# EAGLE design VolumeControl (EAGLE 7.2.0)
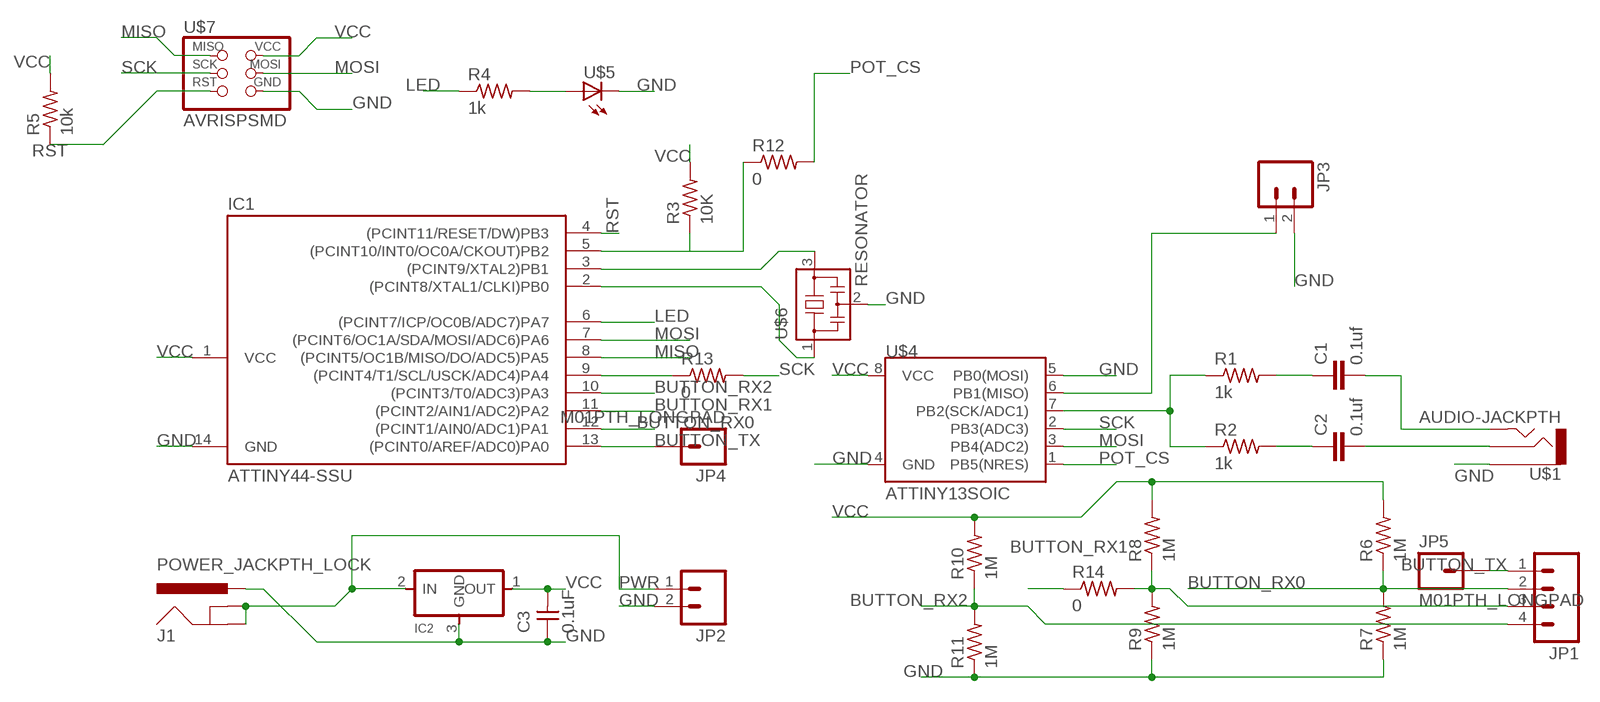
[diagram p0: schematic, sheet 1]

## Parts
C1  0.1uf  CAP1206  [1206]
C2  0.1uf  CAP1206  [1206]
C3  0.1uF  UNPOLARIZED_CAPACITOR1206  [1206]
IC1  ATTINY44-SSU  [SOIC14]
IC2  REGULATORSOT23  [SOT23]
J1  POWER_JACKPTH_LOCK  [POWER_JACK_PTH_LOCK]
JP1  M04SMD  [1X04-SMD]
JP2  M02LOCK_LONGPADS  [1X02_LOCK_LONGPADS]
JP3  M02LOCK_LONGPADS  [1X02_LOCK_LONGPADS]
JP4  M01PTH_LONGPAD  [1X01_LONGPAD]
JP5  M01PTH_LONGPAD  [1X01_LONGPAD]
R1  1k  RESISTOR1206  [1206]
R2  1k  RESISTOR1206  [1206]
R3  10K  RESISTOR1206  [1206]
R4  1k  RESISTOR1206  [1206]
R5  10k  RESISTOR1206  [1206]
R6  1M  RESISTOR1206  [1206]
R7  1M  RESISTOR1206  [1206]
R8  1M  RESISTOR1206  [1206]
R9  1M  RESISTOR1206  [1206]
R10  1M  RESISTOR1206  [1206]
R11  1M  RESISTOR1206  [1206]
R12  0  RESISTOR1206  [1206]
R13  0  RESISTOR1206  [1206]
R14  0  RESISTOR1206  [1206]
U$1  AUDIO-JACKPTH  [AUDIO-JACK]
U$4  ATTINY13SOIC  [SO08]
U$5  LED1206  [1206]
U$6  RESONATOR  [EFOBM]
U$7  AVRISPSMD  [2X03SMD]

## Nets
BUTTON_RX0: IC1.12((PCINT1/AIN0/ADC1)PA1) JP1.2 R6.1 R7.2
BUTTON_RX1: IC1.11((PCINT2/AIN1/ADC2)PA2) JP1.3 R8.1 R9.2 R14.1 R14.2
BUTTON_RX2: IC1.10((PCINT3/T0/ADC3)PA3) JP1.4 R10.1 R11.2
BUTTON_TX: IC1.13((PCINT0/AREF/ADC0)PA0) JP1.1 JP4.1 JP5.1
GND: C3.1 IC1.14(GND) IC2.3(GND) J1.PWR JP2.2 JP3.2 R7.1 R9.1 R11.1 U$1.1 U$4.4(GND) U$4.5(PB0(MOSI)) U$5.2(C) U$6.2 U$7.6(GND)
LED: IC1.6((PCINT7/ICP/OC0B/ADC7)PA7) R4.1
MISO: IC1.8((PCINT5/OC1B/MISO/DO/ADC5)PA5) U$7.1(MISO)
MOSI: IC1.7((PCINT6/OC1A/SDA/MOSI/ADC6)PA6) U$4.3(PB4(ADC2)) U$7.4(MOSI)
N$8: C2.2 U$1.2
N$9: C1.2 U$1.5
N$10: C1.1 R1.2
N$11: C2.1 R2.2
N$12: R1.1 R2.1 U$4.7(PB2(SCK/ADC1))
N$13: JP3.1 U$4.6(PB1(MISO))
N$14: R4.2 U$5.1(A)
N$15: IC1.3((PCINT9/XTAL2)PB1) U$6.3
N$16: IC1.2((PCINT8/XTAL1/CLKI)PB0) U$6.1
POT_CS: IC1.5((PCINT10/INT0/OC0A/CKOUT)PB2) R3.1 R12.1 R12.2 U$4.1(PB5(NRES))
PWR: IC2.2(IN) J1.GND J1.GNDBREAK JP2.1
RST: IC1.4((PCINT11/RESET/DW)PB3) R5.1 U$7.5(RST)
SCK: IC1.9((PCINT4/T1/SCL/USCK/ADC4)PA4) R13.1 R13.2 U$4.2(PB3(ADC3)) U$7.3(SCK)
VCC: C3.2 IC1.1(VCC) IC2.1(OUT) R3.2 R5.2 R6.2 R8.2 R10.2 U$4.8(VCC) U$7.2(VCC)

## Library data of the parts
C1 C2 = 01_SparkFun:CAP: Capacitor
C3 = 01_ng:UNPOLARIZED_CAPACITOR: unpolarized_capacitor
IC1 = 01_fab:ATTINY44
IC2 = 01_fab:REGULATOR
J1 = 01_SparkFun:POWER_JACK: Power Jack This is the standard 5.5mm barrel jack for power. The PTH is the most common, proven, reliable, footprint. All others are experimental. The Slot footprint only works if the mill layer is transmitted to the PCB fab house so be warned. Spark Fun Electronics SKU : PRT-00119. Mating wall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
JP1 = 01_SparkFun:M04: Header 4 Standard 4-pin 0.1" header. Use with straight break away headers (SKU : PRT-00116), right angle break away headers (PRT-00553), swiss pins (PRT-00743), machine pins (PRT-00117), and female headers (PRT-00115). Molex polarized connector foot print use with SKU : PRT-08231 with associated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
JP2 JP3 = 01_SparkFun:M02: Header 2
JP4 JP5 = 01_SparkFun:M01: Header 1
R1-R14 = 01_FAB_Hello:RESISTOR
U$1 = 01_SparkFun:AUDIO-JACK: 3.5mm Audio Jack Simple 3.5mm common PCB mount audio jack. SKU: PRT-08032
U$4 = 01_SparkFun:ATTINY13
U$5 = 01_FAB_Hello:LED
U$6 = 01_fab:RESONATOR
U$7 = 01_fab:AVRISP

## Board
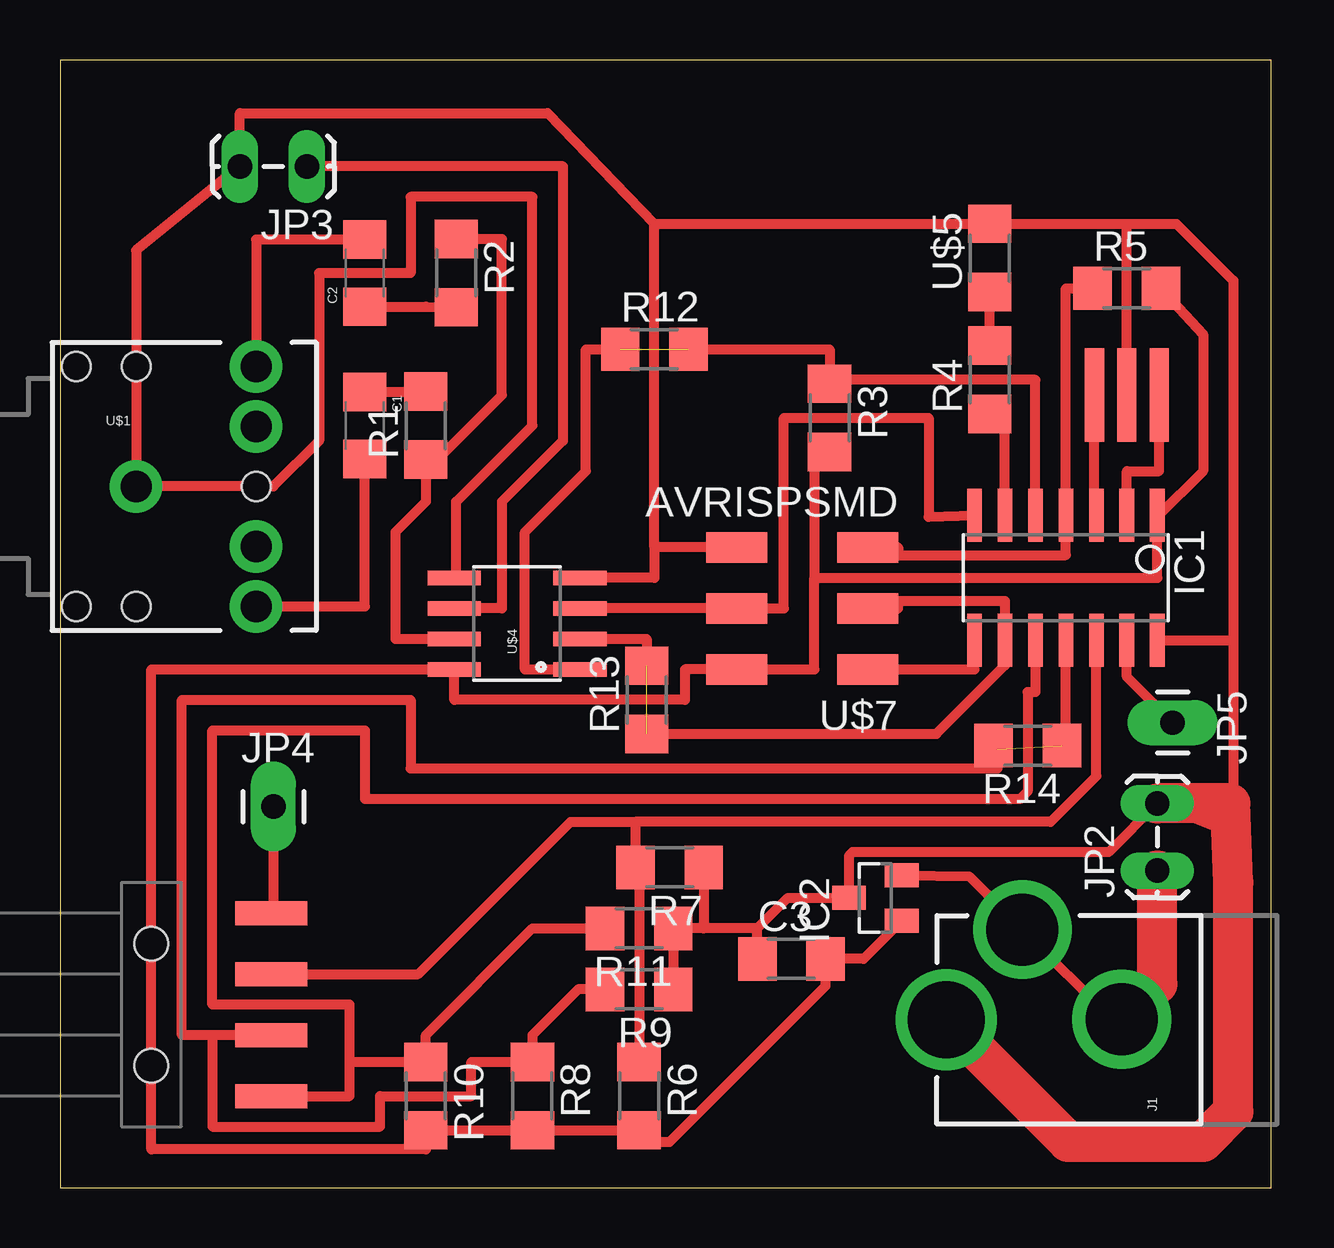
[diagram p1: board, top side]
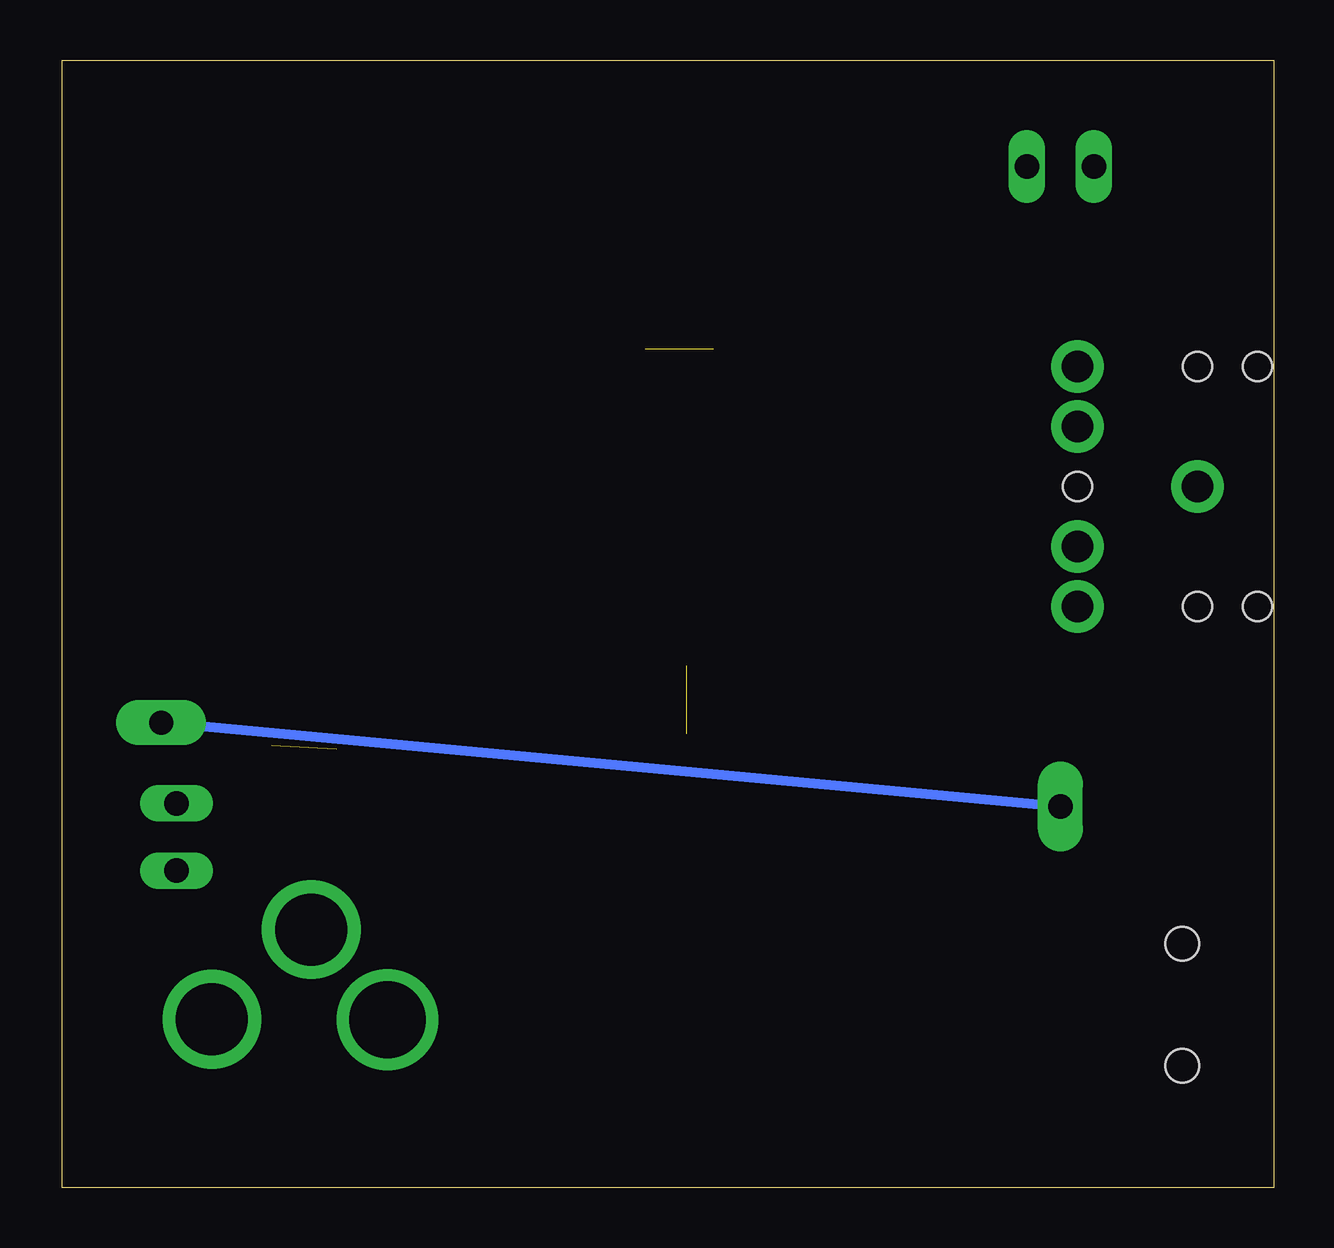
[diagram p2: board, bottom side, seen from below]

Size 50.47 x 46.98 mm. Coordinates in mm from the lower left corner, seen from the top.
Outline: 0,0 50.47,0 50.47,46.98 0,46.98 0,0
Copper layers (1*16): Top 0.035mm / dielectric 1.5mm / Bottom 0.035mm
Design rules "default": minimum track width 10mil, minimum drill 24mil, track to track 8mil, track to pad 8mil, pad to pad 8mil, via to via 8mil, smd to smd 8mil, copper to edge 40mil, drill to drill 8mil, minimum pad ring 10mil, minimum via ring 8mil, stop-mask expansion 4mil, vias tented up to drill 0mil, thermal gap 10mil

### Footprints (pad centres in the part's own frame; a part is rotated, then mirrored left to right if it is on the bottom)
1206 = smd 1.6 x 1.8: 1 -1.4,0; 2 1.4,0
1206' = smd 1.6 x 1.803: 1 -1.422,0; 2 1.422,0
SOIC14 = smd 0.61 x 2.21: 1 -3.81,-2.603; 2 -2.54,-2.603; 3 -1.27,-2.603; 4 0,-2.603; 5 1.27,-2.603; 6 2.54,-2.603; 7 3.81,-2.603; 8 3.81,2.603; 9 2.54,2.603; 10 1.27,2.603; 11 0,2.603; 12 -1.27,2.603; 13 -2.54,2.603; 14 -3.81,2.603
SOT23 = smd 1 x 1.4: 1 -0.95,-1.1; 2 0.95,-1.1; 3 0,1.1
POWER_JACK_PTH_LOCK = drill 2.997 pad 4.115: GND 0.025,6.557; GNDBREAK 3.762,10.7 | drill 3.2 pad 4.115: PWR 0,13.878
1X04-SMD = smd 1 x 3: 1 -3.81,5; 2 -1.27,5; 3 1.27,5; 4 3.81,5 | hole 1.4: -2.54,0; 2.54,0
1X02_LOCK_LONGPADS = drill 1.016 long: 1 -0.127,0; 2 2.667,0
1X01_LONGPAD = drill 1.016 pad 1.88 long: 1 0,0
AUDIO-JACK = drill 1.3 pad 2.184: 1 0,0; 2 5,5; 3 5,2.5; 4 5,-2.5; 5 5,-5 | hole 1.2: 0,5; -2.5,5; -2.5,-5; 0,-5; 5,0
SO08 = smd 0.61 x 2.21: 1 -1.905,-2.616; 2 -0.635,-2.616; 3 0.635,-2.616; 4 1.905,-2.616; 5 1.905,2.616; 6 0.635,2.616; 7 -0.635,2.616; 8 -1.905,2.616
EFOBM = smd 0.8 x 3.9: 1 -1.35,0; 2 0,0; 3 1.35,0
2X03SMD = smd 2.54 x 1.27: 1 -2.54,2.54; 2 2.92,2.54; 3 -2.54,0; 4 2.92,0; 5 -2.54,-2.54; 6 2.92,-2.54

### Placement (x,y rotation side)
C1  12.7,31.75 270 top
C2  12.7,38.1 90 top
C3  0.1uF  [1206']  30.48,9.53 0 top
IC1  41.91,25.4 180 top
IC2  33.97,12.06 90 top
J1  50.8,6.99 90 top
JP1  3.81,7.62 270 top
JP2  45.72,13.34 90 top
JP3  10.16,42.55 180 top
JP4  8.89,15.88 0 top
JP5  46.35,19.37 270 top
R1  1k  [1206']  15.24,31.75 90 top
R2  1k  [1206']  16.51,38.1 270 top
R3  10K  [1206']  32.07,32.07 270 top
R4  1k  [1206']  38.73,33.66 90 top
R5  10k  [1206']  44.45,37.47 0 top
R6  1M  [1206']  24.13,3.81 270 top
R7  1M  [1206']  25.4,13.34 180 top
R8  1M  [1206']  19.68,3.81 270 top
R9  1M  [1206']  24.13,8.26 180 top
R10  1M  [1206']  15.24,3.81 270 top
R11  1M  [1206']  24.13,10.79 180 top
R12  0  [1206']  24.77,34.92 0 top
R13  0  [1206']  24.45,20.32 90 top
R14  0  [1206']  40.32,18.41 180 top
U$1  3.17,29.21 0 top
U$4  19.05,23.5 90 top
U$5  [1206']  38.73,38.73 90 top
U$6  44.45,33.02 180 top
U$7  31.11,24.13 180 top

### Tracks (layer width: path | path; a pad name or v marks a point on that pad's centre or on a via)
BUTTON_RX0
  Top 0.406: JP1.2 14.92,8.89 21.27,15.24 23.98,15.24 | 23.98,15.24 R7.2 24.13,13.18 R6.1 | 23.98,15.24 41.27,15.24 43.18,17.14 IC1.12
BUTTON_RX1  (1 unrouted)
  Top 0.406: JP1.3 6.35,6.35 | 6.35,6.35 6.35,2.54 13.34,2.54 13.34,3.81 17.14,3.81 17.14,5.23 R8.1 19.68,6.35 21.59,8.26 R9.2 | 6.35,6.35 5.08,6.35 5.08,20.32 14.61,20.32 14.61,17.46 39.05,17.46 39.05,18.26 R14.2 | R14.1 41.91,18.58 IC1.11
BUTTON_RX2
  Top 0.406: JP1.4 12.06,3.81 12.06,5.23 | 12.06,5.23 R10.1 15.24,6.35 19.68,10.79 R11.2 | 12.06,5.23 12.06,7.62 6.35,7.62 6.35,19.05 12.7,19.05 12.7,16.19 40.01,16.19 40.32,16.51 40.32,20.64 40.64,20.64 IC1.10
BUTTON_TX
  Top 0.406: JP4.1 8.89,11.43 JP1.1 | JP5.1 44.45,21.27 IC1.13
  Bottom 0.406: JP4.1 JP5.1
GND
  Top 0.406: U$7.6 24.77,26.67 | 24.77,26.67 24.77,25.4 U$4.4 | U$6.2 44.45,40.16 | 48.9,22.8 48.9,37.78 46.52,40.16 44.45,40.16 | 48.9,22.8 48.9,14.73 JP2.2 43.69,13.97 33.02,13.97 32.87,13.82 IC2.3 30.33,12.06 29.06,10.79 | 44.45,40.16 U$5.2 24.77,40.16 | U$4.5 16.51,25.48 16.51,28.57 19.68,31.75 19.68,41.27 14.61,41.27 14.61,38.1 10.79,38.1 10.79,31.11 8.89,29.21 U$1.1 3.17,39.05 JP3.2 7.49,44.77 20.32,44.77 24.77,40.16 | 24.77,26.67 24.77,40.16 | IC1.14 48.9,22.8 | R9.1 R11.1 26.82,10.79 | R7.1 26.82,10.79 | C3.1 29.06,10.79 | 29.06,10.79 26.82,10.79
  Top 1.676: J1.PWR 42,1.91 47.62,1.91 48.9,3.17 48.9,12.7 48.77,16 JP2.2
LED
  Top 0.406: IC1.6 39.37,32.23 R4.1
MISO
  Top 0.406: U$7.1 38.1,21.59 IC1.8
MOSI
  Top 0.406: IC1.7 36.2,27.94 36.2,32.07 30.16,32.07 30.16,24.13 U$7.4 U$4.3
N$8
  Top 0.406: C2.2 8.18,39.5 U$1.2
N$9
  Top 0.406: U$1.5 12.7,24.21 C1.2
N$10
  Top 0.406: C1.1 15.24,33.15 R1.2
N$11
  Top 0.406: C2.1 15.24,36.7 R2.2
N$12
  Top 0.406: R2.1 18.41,39.52 18.41,33.02 15.88,30.48 15.24,30.48 R1.1 15.24,28.57 13.97,27.3 13.97,22.86 U$4.7
N$13
  Top 0.406: U$4.6 18.41,24.13 18.41,28.57 20.95,31.11 20.95,42.55 JP3.1
N$14
  Top 0.406: R4.2 U$5.1
N$15
  Top 0.406: IC1.3 43.1,28 U$6.3
N$16
  Top 0.406: IC1.2 44.45,29.84 45.8,29.84 U$6.1
POT_CS  (1 unrouted)
  Top 0.406: IC1.5 40.64,33.66 31.43,33.66 R3.1 32.07,34.92 R12.2 | U$4.1 19.37,21.59 19.37,27.3 21.91,29.84 21.91,34.92 R12.1
PWR
  Top 0.406: IC2.2 37.88,12.97 J1.GNDBREAK 43.84,7.01 J1.GND
  Top 1.676: J1.GND 45.72,8.49 JP2.1
RST
  Top 0.406: U$7.5 34.92,26.67 34.92,26.35 41.91,26.35 IC1.4 41.91,37.47 R5.1
SCK  (1 unrouted)
  Top 0.406: U$7.3 34.92,24.13 34.92,24.45 39.37,24.45 IC1.9 39.37,21.76 36.51,18.9 R13.1 | U$4.2 24.45,22.86 R13.2
VCC
  Top 0.406: 31.43,25.4 31.43,21.59 U$7.2 26.04,21.59 26.04,20.32 16.43,20.32 U$4.8 3.81,21.59 3.81,1.59 15.24,1.59 R10.2 R8.2 R6.2 24.13,1.91 25.4,1.91 31.9,8.41 C3.2 33.49,9.53 IC2.1 | 31.43,25.4 45.72,25.4 45.72,27.94 | R5.2 47.62,35.56 47.62,29.84 45.72,27.94 | 45.72,27.94 IC1.1 | R3.2 31.43,30.64 31.43,25.4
